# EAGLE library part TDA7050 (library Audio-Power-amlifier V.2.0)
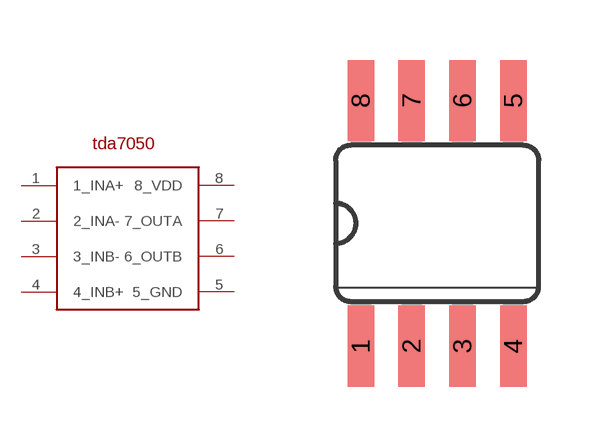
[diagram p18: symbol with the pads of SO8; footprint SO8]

Designator prefix -

## TDA7050SO8  [SO8]
1  1_INA+
2  2_INA-
3  3_INB-
4  4_INB+
5  5_GND
6  6_OUTB
7  7_OUTA
8  8_VDD

## Footprint SO8 (pad centres in mm)
smd 0.66 x 2.032: 1 -1.905,-3.073; 2 -0.635,-3.073; 3 0.635,-3.073; 4 1.905,-3.073; 5 1.905,3.073; 6 0.635,3.073; 7 -0.635,3.073; 8 -1.905,3.073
